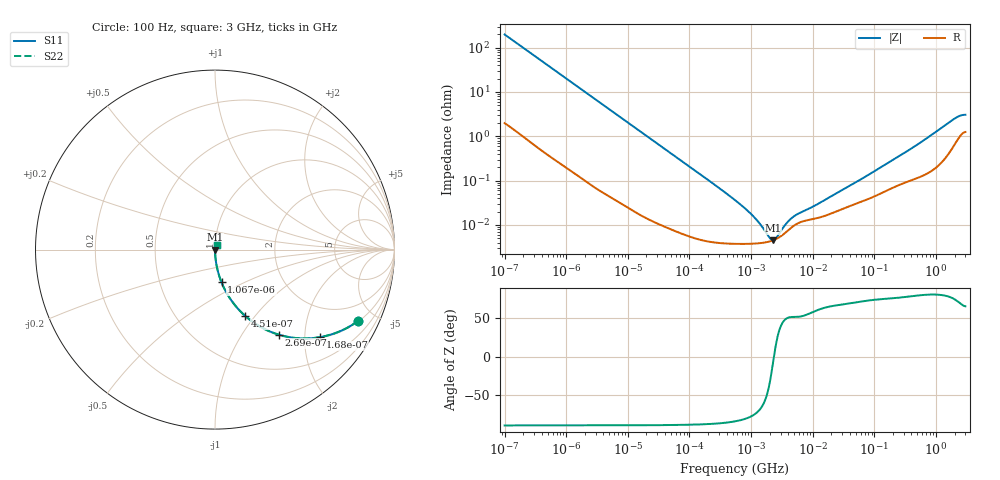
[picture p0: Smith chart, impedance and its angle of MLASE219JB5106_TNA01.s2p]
! MLASE219JB5106_TNA01  S-PARAMETER MODEL  ( Standard Model )
! Model Generated by TAIYO YUDEN Corporation (http://www.ty-top.com)
! Version 1.0
! TAIYO YUDEN Control No. 220601
! Copyright(c) 2009 TAIYO YUDEN CO.,LTD. All Rights Reserved.
! Product Description (link to TY-COMPAS)
! https://ds.yuden.co.jp/TYCOMPAS/or/detail?pn=MLASE219JB5106KTNA01&u=M
! Products Name : Multilayer Ceramic Capacitors
! Characteristics :
!  Capacitance : 10 [uF] , Rated Voltage : 16 [V] , TCC : X5R
!  Case Size : 2.0 x 1.25 / 0.079 x 0.049 [mm/inch] , Thickness : 0.85 / 0.033 [mm/inch]
!  (Conditions: Temperature = 25 [degC] , DC Bias Voltage = 0 [V])
! External Node Assignments :
!  1  o---| |---o  2
! GND o---------o GND
! Frequency Range : 100Hz  -  3GHz  [ 401 STEP ]
# MHZ S RI R 50
! Freq[MHz].  S11 Real  S11 Imag  S21 Real  S21 Imag  S12 Real  S12 Imag  S22 Real  S22 Imag
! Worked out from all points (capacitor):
!   401 points, 100 Hz to 3 GHz, reference 50 ohm
!   read as one part in series: C = 7.98 uF near 109 Hz
!   lowest |Z| = 4.53 mohm at 2.267 MHz (marker M1)
!   series resonance near 2.345 MHz, so ESL is about 580 pH
!   S11 on the Smith chart (normalised r, x): 100 Hz: 1.04, -3.98; 168 Hz: 1.02, -2.38; 269 Hz: 1.01, -1.49; 451 Hz: 1.01, -0.89; 1.067 kHz: 1.00, -0.38; 3 GHz: 1.03, +0.06
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0.0001  0.7961 -0.3979  0.2039 0.3979  0.2039 0.3979  0.7961 -0.3979
0.000168  0.5861 -0.4876  0.4139 0.4876  0.4139 0.4876  0.5861 -0.4876
0.000269  0.3581 -0.4746  0.6419 0.4746  0.6419 0.4746  0.3581 -0.4746
0.000451  0.168 -0.3692  0.832 0.3692  0.832 0.3692  0.168 -0.3692
0.000664  0.0864 -0.2762  0.9136 0.2762  0.9136 0.2762  0.0864 -0.2762
0.001067  0.0363 -0.1822  0.9637 0.1822  0.9637 0.1822  0.0363 -0.1822
0.001788  0.0138 -0.1117  0.9862 0.1117  0.9862 0.1117  0.0138 -0.1117
0.005476  0.00179 -0.0372  0.9982 0.0372  0.9982 0.0372  0.00179 -0.0372
0.031977  0.000145 -0.00645  0.9999 0.00645  0.9999 0.00645  0.000145 -0.00645
0.547723  3.76e-05 -0.000362  1 0.000362  1 0.000362  3.76e-05 -0.000362
0.918067  3.75e-05 -0.000194  1 0.000194  1 0.000194  3.75e-05 -0.000194
1.411895  3.89e-05 -9.55e-05  1 9.55e-05  1 9.55e-05  3.89e-05 -9.55e-05
1.6065  3.98e-05 -7e-05  1 7e-05  1 7e-05  3.98e-05 -7e-05
2.266852  4.49e-05 -6.09e-06  1 6.09e-06  1 6.09e-06  4.49e-05 -6.09e-06
3.486191  6.44e-05 7.11e-05  0.9999 -7.11e-05  0.9999 -7.11e-05  6.44e-05 7.11e-05
5.361412  0.000103 0.000133  0.9999 -0.000133  0.9999 -0.000133  0.000103 0.000133
9.794414  0.000135 0.000215  0.9999 -0.000215  0.9999 -0.000215  0.000135 0.000215
175.1444  0.000642 0.00254  0.9994 -0.00254  0.9994 -0.00254  0.000642 0.00254
513.708  0.00121 0.00658  0.9988 -0.00658  0.9988 -0.00658  0.00121 0.00658
2036.508  0.0073 0.0242  0.9927 -0.0242  0.9927 -0.0242  0.0073 0.0242
2525.516  0.0112 0.027  0.9888 -0.027  0.9888 -0.027  0.0112 0.027
3000  0.0131 0.0273  0.9869 -0.0273  0.9869 -0.0273  0.0131 0.0273
